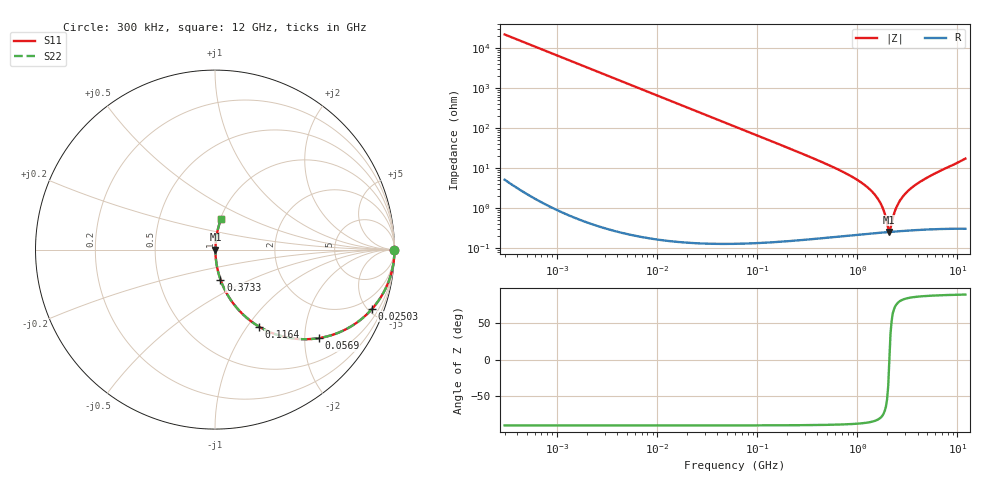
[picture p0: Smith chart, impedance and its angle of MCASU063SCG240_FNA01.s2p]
! MCASU063SCG240_FNA01  S-PARAMETER MODEL  ( General Type )
! Model Generated by TAIYO YUDEN Corporation (http://www.ty-top.com)
! Version 1.0
! TAIYO YUDEN Control No. 130801
! Copyright(c) 2013 TAIYO YUDEN CO.,LTD. All Rights Reserved.
! Product Description (link to TY-COMPAS)
! https://ds.yuden.co.jp/TYCOMPAS/or/detail?pn=MCASU063SCG240JFNA01&u=M
! Products Name : Multilayer Ceramic Capacitors
! Characteristics :
!  Capacitance : 24 pF , Rated Voltage : 50V , TCC : CG / C0G
!  Case Size : 0.6 x 0.3 / 0.024 x 0.012 [mm/inch] , Thickness : 0.3 / 0.012 [mm/inch]
!  (Conditions: Temperature = 25 degC , DC Bias Current/Voltage = 0A / 0V)
! External Node Assignments :
!  1  o---| |---o  2
! GND o---------o GND
! Frequency Range : 0.3MHz  -  12000MHz  [ 401 STEP ]
# MHz S RI R 50
! Freq[MHz].  S11 Real  S11 Imag  S21 Real  S21 Imag  S12 Real  S12 Imag  S22 Real  S22 Imag
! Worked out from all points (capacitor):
!   401 points, 300 kHz to 12 GHz, reference 50 ohm
!   read as one part in series: C = 23.9 pF near 316.3 kHz
!   lowest |Z| = 257 mohm at 2.089 GHz (marker M1)
!   series resonance near 2.087 GHz, so ESL is about 240 pH
!   S11 on the Smith chart (normalised r, x): 300 kHz: open; 25.03 MHz: 1.00, -5.33; 56.9 MHz: 1.00, -2.34; 116.4 MHz: 1.00, -1.14; 373.3 MHz: 1.00, -0.35; 12 GHz: 1.01, +0.35
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0.3  1 -0.0045  2.13e-05 0.0045  2.13e-05 0.0045  1 -0.0045
1.769972  0.9993 -0.0265  0.000708 0.0265  0.000708 0.0265  0.9993 -0.0265
10.44266  0.976 -0.1528  0.024 0.1528  0.024 0.1528  0.976 -0.1528
25.03118  0.8763 -0.3289  0.1237 0.3289  0.1237 0.3289  0.8763 -0.3289
56.90376  0.5782 -0.4933  0.4218 0.4933  0.4218 0.4933  0.5782 -0.4933
60  0.5521 -0.4967  0.4479 0.4967  0.4479 0.4967  0.5521 -0.4967
116.3536  0.2466 -0.4298  0.7534 0.4298  0.7534 0.4298  0.2466 -0.4298
192.4766  0.1066 -0.3064  0.8934 0.3064  0.8934 0.3064  0.1066 -0.3064
353.9943  0.0339 -0.1765  0.9661 0.1765  0.9661 0.1765  0.0339 -0.1765
373.2558  0.0306 -0.1674  0.9694 0.1674  0.9694 0.1674  0.0306 -0.1674
804.7407  0.007 -0.07  0.993 0.07  0.993 0.07  0.007 -0.07
1296.429  0.00331 -0.0315  0.9967 0.0315  0.9967 0.0315  0.00331 -0.0315
1689.663  0.00264 -0.0137  0.9974 0.0137  0.9974 0.0137  0.00264 -0.0137
1829.429  0.00257 -0.0086  0.9974 0.0086  0.9974 0.0086  0.00257 -0.0086
1980.756  0.00255 -0.00354  0.9974 0.00354  0.9974 0.00354  0.00255 -0.00354
2088.533  0.00257 4.8e-05  0.9974 -4.8e-05  0.9974 -4.8e-05  0.00257 4.8e-05
2202.174  0.00261 0.00344  0.9974 -0.00344  0.9974 -0.00344  0.00261 0.00344
2384.334  0.00271 0.00841  0.9973 -0.00841  0.9973 -0.00841  0.00271 0.00841
2581.562  0.00285 0.0133  0.9971 -0.0133  0.9971 -0.0133  0.00285 0.0133
3364.605  0.00371 0.0301  0.9963 -0.0301  0.9963 -0.0301  0.00371 0.0301
5278.635  0.00696 0.0629  0.993 -0.0629  0.993 -0.0629  0.00696 0.0629
12000  0.0326 0.169  0.9674 -0.169  0.9674 -0.169  0.0326 0.169
